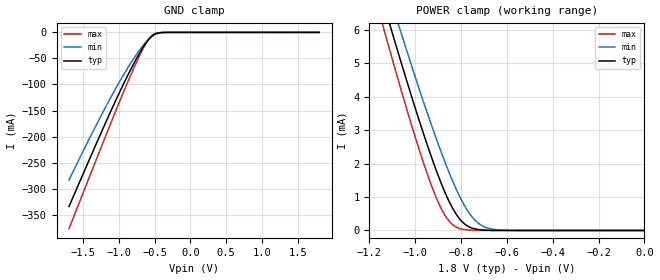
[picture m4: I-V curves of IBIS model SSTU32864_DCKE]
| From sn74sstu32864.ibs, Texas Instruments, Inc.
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[Model]   SSTU32864_DCKE
Model_type  Input
Vinl=0.844
Vinh=0.958
| variable   typ   min   max
C_comp   2.09pF   1.67pF   2.27pF
[Temperature Range]   40   85   0
| Ambient temperature   25   70   0
[Voltage range]   1.8   1.7   1.9
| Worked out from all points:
|   GND clamp passes 1 mA (typ) near -0.45 V on its own axis
|   POWER clamp passes 1 mA (typ) near -0.86 V on its own axis
[GND Clamp]
| SSTU32864_DCKE
|   Voltage   I(typ)   I(min)   I(max)
-1.7V     -334.4mA   -283.3mA   -376.9mA
-1.28V    -201.8mA   -167.7mA   -230.9mA
-970mV    -108.4mA   -89.28mA   -125.4mA
-815mV    -65.51mA   -54.47mA   -75.34mA
-685mV    -33.41mA   -29mA      -36.76mA
-605mV    -16.88mA   -15.99mA   -17mA
-535mV    -6.576mA   -7.343mA   -5.649mA
-460mV    -1.429mA   -2.103mA   -934.7uA
-340mV    -49.41uA   -124uA     -18.04uA
1.8V      1.074nA    8.658nA    119.1pA
[POWER Clamp]
| SSTU32864_DCKE
|   Voltage   I(typ)   I(min)   I(max)
-1.7V     20.54mA    20.56mA    20.57mA
-1.14V    6.837mA    7.627mA    6.099mA
-1.1V     5.907mA    6.744mA    5.124mA
-1.06V    4.993mA    5.872mA    4.169mA
-980mV    3.235mA    4.179mA    2.363mA
-915mV    1.926mA    2.879mA    1.097mA
-865mV    1.061mA    1.956mA    400.2uA
-820mV    474.7uA    1.221mA    98.68uA
-785mV    198uA      747uA      26uA
-745mV    57.1uA     352.4uA    5.154uA
-670mV    4.139uA    49.18uA    235.7nA
-14.28fV  1.074nA    8.252nA    134.1pA
